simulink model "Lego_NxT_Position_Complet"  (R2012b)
settings: Solver=ode45  StartTime=0.0  StopTime=10  RelTol=1e-3
libraries: simulink x1

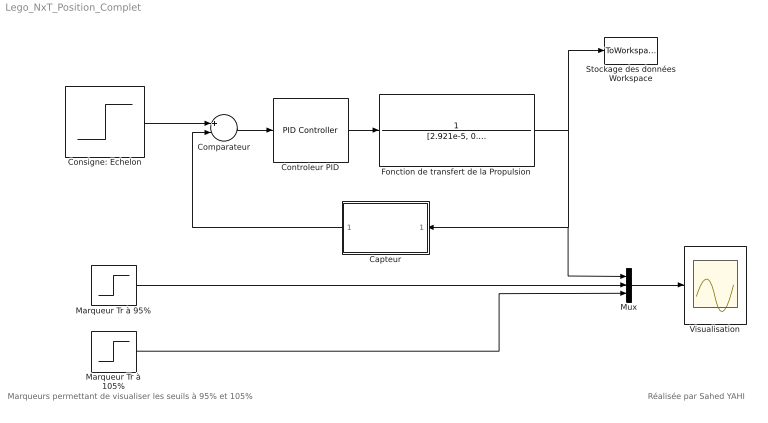
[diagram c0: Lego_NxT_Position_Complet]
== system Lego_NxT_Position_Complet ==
  note: Marqueurs permettant de visualiser les seuils à 95% et 105%
  note: Réalisée par Sahed YAHI
  Capteur : Subsystem
  Comparateur : Sum  Inputs=+-
  Consigne: Echelon : Step  Time=0  After=90  SampleTime=0
  Controleur PID : simulink/Continuous/PID Controller  Controller=PID  TimeDomain=Continuous-time  SampleTime=1  IntegratorMethod=Forward Euler  FilterMethod=Forward Euler  Form=Parallel  P=5  I=50  D=0  N=100  InitialConditionSource=internal  InitialConditionForIntegrator=0  InitialConditionForFilter=0  ExternalReset=none  LimitOutput=off  UpperSaturationLimit=inf  LowerSaturationLimit=-inf  LinearizeAsGain=on  AntiWindupMode=none  Kb=1  TrackingMode=off  Kt=1  PParamMin=[]  PParamMax=[]  IParamMin=[]  IParamMax=[]  DParamMin=[]  DParamMax=[]  NParamMin=[]  NParamMax=[]  KbParamMin=[]  KbParamMax=[]  KtParamMin=[]  KtParamMax=[]  POutMin=[]  POutMax=[]  IOutMin=[]  IOutMax=[]  DOutMin=[]  DOutMax=[]  NOutMin=[]  NOutMax=[]  KbOutMin=[]  KbOutMax=[]  KtOutMin=[]  KtOutMax=[]  IntegratorOutMin=[]  IntegratorOutMax=[]  FilterOutMin=[]  FilterOutMax=[]  SumOutMin=[]  SumOutMax=[]  SumI1OutMin=[]  SumI1OutMax=[]  SumI2OutMin=[]  SumI2OutMax=[]  SumI3OutMin=[]  SumI3OutMax=[]  SumDOutMin=[]  SumDOutMax=[]  SaturationOutMin=[]  SaturationOutMax=[]  IntegratorContinuousStateAttributes=''  IntegratorStateMustResolveToSignalObject=off  IntegratorRTWStateStorageClass=Auto  FilterContinuousStateAttributes=''  FilterStateMustResolveToSignalObject=off  FilterRTWStateStorageClass=Auto
  Fonction de transfert de la Propulsion : TransferFcn  Numerator=1  Denominator=[2.921e-5, 0.0315, 0.5048, 0]
  Marqueur Tr à 105% : Step  Time=0  After=90*1.05  SampleTime=0
  Marqueur Tr à 95% : Step  Time=0  After=90*0.95  SampleTime=0
  Mux : Mux  Inputs=3
  Stockage des données Workspace : ToWorkspace  VariableName=simData  SampleTime=-1  SaveFormat=Timeseries
  Visualisation : Scope
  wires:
  Consigne: Echelon/1 -> Comparateur/1
  Comparateur/1 -> Controleur PID/1
  Capteur/1(Out1) -> Comparateur/2
  Controleur PID/1 -> Fonction de transfert de la Propulsion/1
  Fonction de transfert de la Propulsion/1 -> Capteur/1(In1), Mux/1, Stockage des données Workspace/1
  Marqueur Tr à 95%/1 -> Mux/2
  Marqueur Tr à 105%/1 -> Mux/3
  Mux/1 -> Visualisation/1

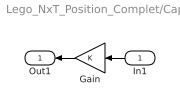
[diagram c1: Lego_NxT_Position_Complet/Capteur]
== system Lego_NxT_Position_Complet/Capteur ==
  In1 : Inport
  Gain : Gain
  Out1 : Outport
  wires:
  In1/1 -> Gain/1
  Gain/1 -> Out1/1
